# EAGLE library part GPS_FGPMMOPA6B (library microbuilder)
FGPMMOPA6B 16x16x0.6mm GPS Module NMEA Sentences: GGA, GSA, GSV, RMC, VTG General Specifications Chipset: MTK MT3329 Baud Rate: 9600bps (default) Update Rate: 1Hz (default) Cold Start: ~35s Operating Temp: -40 to 85°C DC Characteristics Supply Voltage: 3.2-5.0V Backup Battery Voltage: 2.0-4.3V Digital Logic (UART): 3.3V I(Tracking): 42mA I(Acquisition): 53mA I(BackupBattery): 10uA
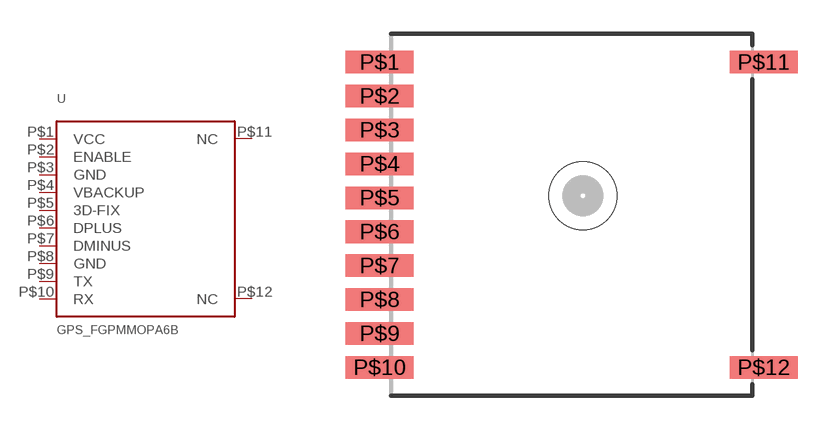
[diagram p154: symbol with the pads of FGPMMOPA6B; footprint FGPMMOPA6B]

Designator prefix U

## GPS_FGPMMOPA6B  [FGPMMOPA6B]
P$1  VCC
P$2  ENABLE
P$3  GND
P$4  VBACKUP
P$5  3D-FIX
P$6  DPLUS
P$7  DMINUS
P$8  GND
P$9  TX
P$10  RX
P$11  NC
P$12  NC

## Footprint FGPMMOPA6B (pad centres in mm)
smd 3 x 1: P$1 -8.5,6.75; P$2 -8.5,5.25; P$3 -8.5,3.75; P$4 -8.5,2.25; P$5 -8.5,0.75; P$6 -8.5,-0.75; P$7 -8.5,-2.25; P$8 -8.5,-3.75; P$9 -8.5,-5.25; P$10 -8.5,-6.75; P$11 8.5,6.75; P$12 8.5,-6.75
hole 3 at 0.5,0.85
